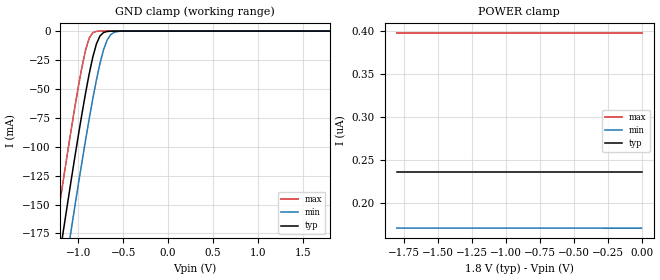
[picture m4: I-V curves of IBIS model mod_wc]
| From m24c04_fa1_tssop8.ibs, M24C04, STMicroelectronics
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|   Model mod_wc
[Model]   mod_wc
Model_type Input
Vinl   =   0.540V
Vinh   =   1.260V
C_comp   1.763pF   1.683pF   1.933pF
[Temperature Range]  25.0000   85.0000   -40.0000
[Voltage Range]   1.8000V   1.7000V   2.0000V
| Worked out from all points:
|   GND clamp passes 1 mA (typ) near -0.71 V on its own axis
[GND_clamp]
|Voltage   I(typ)   I(min)   I(max)
-1.8V     -506.7mA   -549.3mA   -463.8mA
-1.28V    -230.6mA   -274mA     -186.5mA
-1.24V    -209.8mA   -253.3mA   -165.8mA
-1.16V    -168.9mA   -212.2mA   -124.8mA
-1.08V    -128.7mA   -171.8mA   -85.14mA
-920mV    -53.64mA   -94.29mA   -16.44mA
-840mV    -22.68mA   -58.76mA   -1.468mA
-800mV    -11.31mA   -42.6mA    -261.9uA
-720mV    -1.249mA   -16.25mA   -6.98uA
-680mV    -318.6uA   -7.797mA   -1.128uA
-600mV    -18.77uA   -1.043mA   -29.45nA
1.8V      3.674pA    30.76pA    3.627pA
[POWER_clamp]
|Voltage   I(typ)   I(min)   I(max)
-1.8V     235.8nA    170.8nA    397.7nA
-300mV    235.8nA    170.8nA    397.7nA
-280mV    235.8nA    170.7nA    397.7nA
0V        235.8nA    170.7nA    397.7nA
